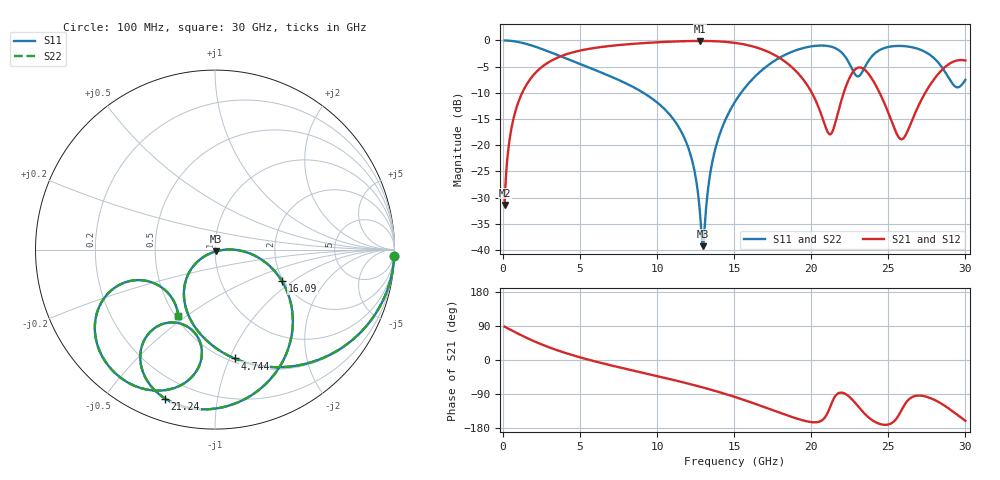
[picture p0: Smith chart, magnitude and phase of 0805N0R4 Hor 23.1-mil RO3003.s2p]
# GHz S MA R 50
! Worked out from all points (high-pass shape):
!   3201 points, 100 MHz to 30 GHz, reference 50 ohm
!   highest |S21| = -0.10 dB at 12.77 GHz (marker M1); lowest = -31.4 dB at 100 MHz (marker M2)
!   |S21| within 3 dB of the highest: 3.679 GHz to 17.81 GHz (14.13 GHz wide, 131 % of centre)
!   lowest |S11| = -39.3 dB at 12.97 GHz (marker M3), VSWR 1.02, Z = 50.3 - j1.05 ohm
!   |S11| at or under -10 dB: 9.106 GHz to 15.44 GHz (6.337 GHz wide, 51.6 % of centre)
!   |S22| runs from -39.3 to 0.0 dB; largest |S21 - S12| = 0
!   S11 on the Smith chart (normalised r, x): 100 MHz: 1, -54; 4.744 GHz: 0.53, -1.04; 16.09 GHz: 1.96, -0.83; 21.24 GHz: 0.10, -0.71; 30 GHz: 0.52, -0.46
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0.1  0.9996 -2.1  0.02688 87.9  0.02688 87.9  0.9996 -2.1
0.5485  0.9893 -11.7  0.1459 78.3  0.1459 78.3  0.9893 -11.7
1.333375  0.9412 -27.7  0.3369 62.3  0.3369 62.3  0.9412 -27.7
4.743844  0.6164 -79.8  0.7845 9.9  0.7845 9.9  0.6164 -79.8
5.089563  0.5882 -83.8  0.8055 5.9  0.8055 5.9  0.5882 -83.8
10.06978  0.2506 -131.7  0.9613 -43.2  0.9613 -43.2  0.2506 -131.7
11.93853  0.1017 -146.5  0.9856 -61.5  0.9856 -61.5  0.1017 -146.5
12.77013  0.02327 -133.8  0.9889 -70.3  0.9889 -70.3  0.02327 -133.8
12.96634  0.01085 -73.7  0.9887 -72.5  0.9887 -72.5  0.01085 -73.7
13.71384  0.08513 0.3  0.9832 -81.0  0.9832 -81.0  0.08513 0.3
15.05  0.2597 -11.6  0.9473 -97.6  0.9473 -97.6  0.2597 -11.6
16.08716  0.4124 -25.2  0.886 -111.8  0.886 -111.8  0.4124 -25.2
18.04934  0.6971 -54.8  0.665 -140.5  0.665 -140.5  0.6971 -54.8
20.03956  0.8794 -87.2  0.3155 -164.1  0.3155 -164.1  0.8794 -87.2
21.24491  0.8751 -108.5  0.1271 -121.5  0.1271 -121.5  0.8751 -108.5
22.19797  0.7004 -126.2  0.347 -89.1  0.347 -89.1  0.7004 -126.2
23.02956  0.4536 -112.2  0.5492 -121.9  0.5492 -121.9  0.4536 -112.2
25.01978  0.868 -116.1  0.2004 -170.0  0.2004 -170.0  0.868 -116.1
25.93547  0.8844 -129.3  0.115 -126.4  0.115 -126.4  0.8844 -129.3
27.43047  0.7715 -149.7  0.3229 -96.6  0.3229 -96.6  0.7715 -149.7
28.79466  0.4694 -158.7  0.5757 -124.5  0.5757 -124.5  0.4694 -158.7
30  0.4204 -119.1  0.6437 -160.3  0.6437 -160.3  0.4204 -119.1
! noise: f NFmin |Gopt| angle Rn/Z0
0.1  0.001812  0.9755  1.543  0.01684
3.417  0.007694  0.7563  22.89  0.006138
6.743  0.013  0.7235  41.17  0.008204
10.06  0.01898  0.7259  58.41  0.01057
13.39  0.02867  0.7629  74.49  0.01572
16.7  0.05463  0.8441  89.82  0.03758
20.03  0.2416  0.9567  104.9  0.4673
23.35  0.2835  0.9579  118.8  0.3943
26.67  0.6175  0.9781  131.9  1.071
30  0.2552  0.942  144.2  0.09378
